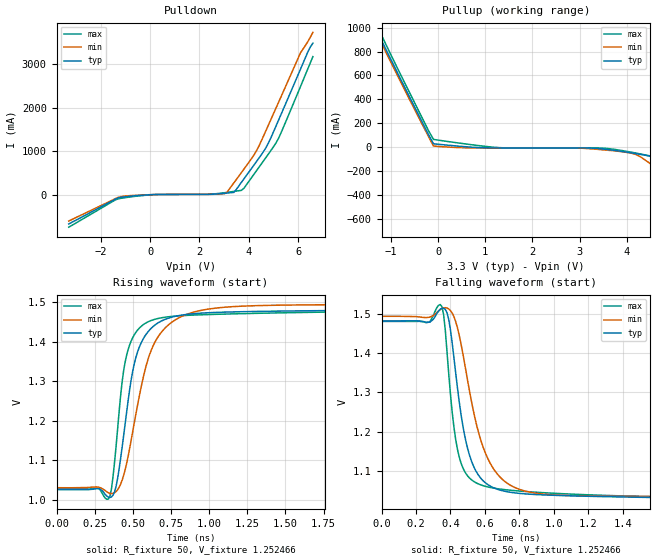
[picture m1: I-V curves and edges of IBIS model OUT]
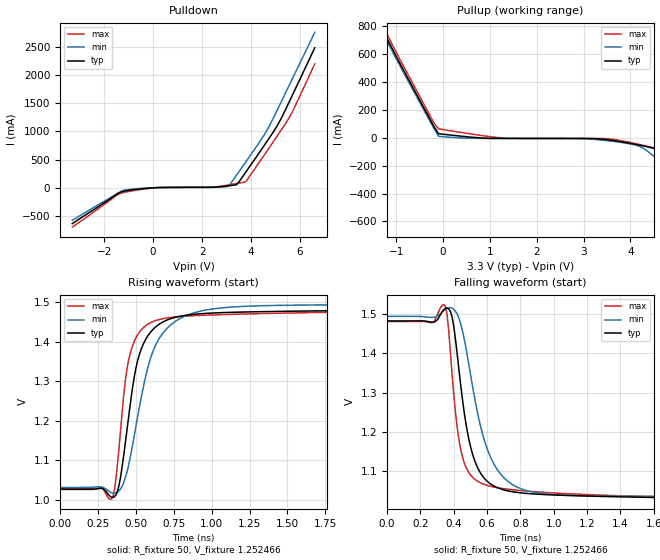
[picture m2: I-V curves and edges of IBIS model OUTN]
|   IBIS File of SG2520VHN C
|   LVDS, Vcc=3.3V, Io=4.5mA, fo<=212.5MHz
[IBIS Ver]   3.2
[File Name]   sg2520vhn_45m_33v.ibs
[File Rev]   1.0
[Date]   Sep. 16, 2020
[Source]
Fairchild Ensigna Lab's Method
[Notes]
Created by Minoru Kozaki
[Disclaimer]
Seiko Epson Corporation makes no warranty with respect to the
information contained herein.
[Copyright]
Copyright(C) 2020, Seiko Epson Corporation. All rights reserved.
|   Component
[Component]   SG2520VHN
[Manufacturer]  Seiko Epson Corporation
[Package]
R_pkg   17.7m   NA   NA
L_pkg   235p   NA   NA
C_pkg   208f   NA   NA
[Pin]   signal_name   model_name   R_pin   L_pin   C_pin
1   OE/ST   NC
2   NC   NC
3   GND   GND
4   OUT   OUT   17.7m   235p   208f
5   OUTN   OUTN   10.4m   129p   221f
6   VCC   POWER
[Diff Pin] inv_pin  vdiff  tdelay_typ
4   5   0   0
| Models and submodels in the file (2): OUT (Output), OUTN (Output)
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|   Model OUT
[Model]   OUT
Model_type   Output
Polarity   Non-Inverting
Vref = 1.25
Vmeas = 1.25
Rref = 50
Cref = 0
C_comp   4.5p   4.5p   4.5p
[Temperature Range]   25   105   -40
[Voltage Range]   3.3   2.97   3.63
[Pullup Reference]   3.3   2.97   3.63
[Pulldown Reference]   0   0   0
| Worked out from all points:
|   slope of the pulldown table from 0 to 0.495 V, typ, clamps not added: 78.1 ohm
|   slope of the pullup table from 0 to 0.495 V, typ, clamps not added: 27.6 ohm
|   falling waveform, R_fixture 50, V_fixture 1.252466: 20-80 % time 109ps typ, 154ps min, 79.7ps max; typ from 1.48 V to 1.03 V
|   rising waveform, R_fixture 50, V_fixture 1.252466: 20-80 % time 123ps typ, 173ps min, 91.6ps max; typ from 1.03 V to 1.48 V
[Pullup]
-3.3V     3.47A      3.398A     3.559A
-1.4V     1.07A      1.064A     1.102A
-1.3V     976mA      959.3mA    1.017A
-1.2V     891.9mA    869mA      934.1mA
-100mV    30.01mA    11.06mA    66.56mA
1.3V      -4.304mA   -4.484mA   -2.324mA
3.2V      -5.386mA   -10.69mA   -4.693mA
4.1V      -45.83mA   -48.62mA   -40.31mA
4.3V      -59.16mA   -80.32mA   -55.6mA
4.6V      -87.91mA   -163.2mA   -80.32mA
5V        -205mA     -274mA     -127.5mA
6.6V      -687.7mA   -707.1mA   -661mA
[Pulldown]
-3.3V     -674.7mA   -607.6mA   -748.4mA
-1.3V     -77.63mA   -64.76mA   -99.38mA
100mV     -812.1uA   -346.2uA   -2.703mA
3.1V      33.3mA     41.14mA    49.67mA
3.4V      50.8mA     272.5mA    73.31mA
3.8V      358.5mA    582mA      142.2mA
4.3V      749.6mA    994.2mA    538.2mA
4.7V      1.081A     1.475A     855mA
5.1V      1.569A     1.983A     1.184A
6.1V      2.886A     3.263A     2.487A
6.4V      3.285A     3.521A     2.897A
6.6V      3.48A      3.729A     3.171A
[Falling Waveform]
R_fixture = 50
V_fixture = 1.252466
V_fixture_min = 1.260431
V_fixture_max = 1.252776
0s        1.483V     1.495V     1.482V
280ps     1.48V      1.492V     1.48V
340ps     1.513V     1.512V     1.525V
370ps     1.512V     1.517V     1.458V
420ps     1.389V     1.494V     1.211V
460ps     1.247V     1.427V     1.121V
570ps     1.084V     1.187V     1.065V
700ps     1.049V     1.078V     1.052V
1.1ns     1.035V     1.036V     1.04V
4ns       1.027V     1.031V     1.028V
[Rising Waveform]
R_fixture = 50
V_fixture = 1.252466
V_fixture_min = 1.260431
V_fixture_max = 1.252776
0s        1.026V     1.031V     1.028V
330ps     1.01V      1.021V     1.002V
370ps     1.012V     1.017V     1.058V
430ps     1.134V     1.05V      1.3V
460ps     1.224V     1.094V     1.367V
530ps     1.373V     1.238V     1.429V
640ps     1.441V     1.396V     1.457V
800ps     1.466V     1.461V     1.466V
1.1ns     1.475V     1.488V     1.47V
4ns       1.483V     1.495V     1.481V
[Ramp]
R_load = 50
dV/dt_r   0.26957/118.64p   0.27301/165.52p   0.26836/88.27p
dV/dt_f   0.26957/107.42p   0.27301/151.73p   0.26836/78.97p
|   Model OUTN
[Model]   OUTN
Model_type   Output
Polarity   Inverting
Vref = 1.25
Vmeas = 1.25
Rref = 50
Cref = 0
C_comp   4.5p   4.5p   4.5p
[Temperature Range]   25   105   -40
[Voltage Range]   3.3   2.97   3.63
[Pullup Reference]   3.3   2.97   3.63
[Pulldown Reference]   0   0   0
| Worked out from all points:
|   slope of the pulldown table from 0 to 0.495 V, typ, clamps not added: 78.4 ohm
|   slope of the pullup table from 0 to 0.495 V, typ, clamps not added: 28 ohm
|   falling waveform, R_fixture 50, V_fixture 1.252466: 20-80 % time 110ps typ, 155ps min, 82.3ps max; typ from 1.48 V to 1.03 V
|   rising waveform, R_fixture 50, V_fixture 1.252466: 20-80 % time 124ps typ, 173ps min, 92.8ps max; typ from 1.03 V to 1.48 V
[Pullup]
-3.3V     2.482A     2.46A      2.508A
-1.4V     840.2mA    821.1mA    872.5mA
-1.3V     775.5mA    756.5mA    806.9mA
-1.2V     711mA      692.6mA    741.6mA
-200mV    82.43mA    69mA       107.8mA
-100mV    29.67mA    11.02mA    65.05mA
1.3V      -4.304mA   -4.484mA   -2.365mA
3.2V      -5.38mA    -10.72mA   -4.693mA
4.1V      -46.18mA   -50.87mA   -40.66mA
4.6V      -87.81mA   -157.9mA   -81.28mA
5V        -196.3mA   -261.9mA   -124.5mA
6.6V      -655.1mA   -679.1mA   -621mA
[Pulldown]
-3.3V     -640.3mA   -581.8mA   -702.9mA
-1.3V     -75.97mA   -63.4mA    -96.78mA
100mV     -829.1uA   -358.2uA   -2.731mA
2.4V      6.168mA    5.593mA    8.003mA
3.1V      32.97mA    32.86mA    49.01mA
3.4V      50.21mA    218.3mA    72.21mA
3.8V      286.1mA    466.4mA    112.9mA
4.6V      790.9mA    983.6mA    617.5mA
5.1V      1.125A     1.409A     940mA
5.5V      1.473A     1.768A     1.204A
5.7V      1.657A     1.948A     1.361A
6.6V      2.486A     2.762A     2.201A
[Falling Waveform]
R_fixture = 50
V_fixture = 1.252466
V_fixture_min = 1.260431
V_fixture_max = 1.252776
0s        1.483V     1.495V     1.481V
340ps     1.511V     1.509V     1.525V
370ps     1.514V     1.517V     1.459V
420ps     1.402V     1.501V     1.214V
460ps     1.258V     1.443V     1.125V
510ps     1.147V     1.323V     1.085V
580ps     1.083V     1.183V     1.066V
700ps     1.051V     1.083V     1.054V
1.1ns     1.037V     1.037V     1.041V
4ns       1.027V     1.032V     1.029V
[Rising Waveform]
R_fixture = 50
V_fixture = 1.252466
V_fixture_min = 1.260431
V_fixture_max = 1.252776
0s        1.027V     1.032V     1.028V
340ps     1.007V     1.018V     1.003V
390ps     1.04V      1.023V     1.139V
430ps     1.144V     1.056V     1.302V
460ps     1.235V     1.103V     1.367V
530ps     1.376V     1.249V     1.428V
640ps     1.441V     1.399V     1.455V
800ps     1.465V     1.461V     1.464V
1.1ns     1.474V     1.487V     1.469V
4ns       1.482V     1.495V     1.481V
[Ramp]
R_load = 50
dV/dt_r   0.26789/118.39p   0.27130/164.20p   0.26668/88.68p
dV/dt_f   0.26789/108.59p   0.27130/151.45p   0.26668/81.02p
